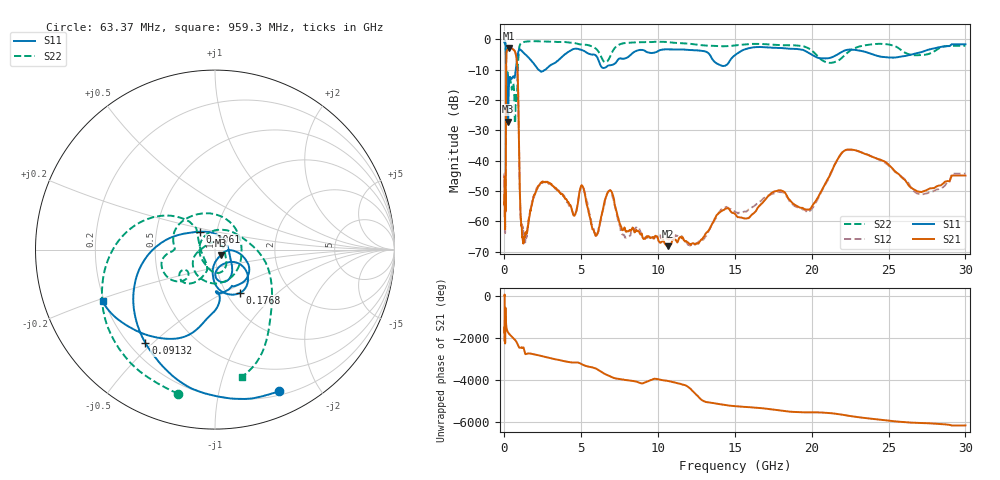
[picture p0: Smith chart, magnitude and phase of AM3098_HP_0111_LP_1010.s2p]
! Date/Time: Thu, Feb 28, 2019 8:39 AM
! Network Analyzer: Agilent Technologies E8364B Rev: A.07.50.67
! Sweep from 0.010 to 30.000 GHz, 1601 Points, Sweep Type: LOG
! Power Supply: 5.022 V, 0.002 A
# Hz S DB R 50
!freq MagS11 AngS11 MagS21 AngS21 MagS12 AngS12 MagS22 AngS22
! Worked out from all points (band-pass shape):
!   1601 points, 10 MHz to 30 GHz, reference 50 ohm
!   highest |S21| = -2.82 dB at 293 MHz (marker M1); lowest = -68.2 dB at 10.65 GHz (marker M2)
!   |S21| within 3 dB of the highest: 121.8 MHz to 773.3 MHz (651.4 MHz wide, 146 % of centre)
!   lowest |S11| = -27.1 dB at 239.9 MHz (marker M3), VSWR 1.09, Z = 53.3 - j3.15 ohm
!   |S11| at or under -10 dB: 102.2 MHz to 730.8 MHz (628.6 MHz wide, 151 % of centre); 2.223 GHz to 2.656 GHz (433.5 MHz wide, 17.8 % of centre)
!   |S22| runs from -27.7 to -0.6 dB; largest |S21 - S12| = 0.01
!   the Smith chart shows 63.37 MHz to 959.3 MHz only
!   S11 on the Smith chart (normalised r, x): 63.37 MHz: 0.24, -1.52; 91.32 MHz: 0.26, -0.47; 106.1 MHz: 0.83, +0.17; 176.8 MHz: 1.15, -0.60; 959.3 MHz: 0.19, -0.21
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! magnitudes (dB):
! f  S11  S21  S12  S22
! 10 MHz  -0.3  -45.2  -44.6  -0.6
! 38.04 MHz  -0.5  -60.3  -59.6  -0.9
! 63.37 MHz  -1.2  -51.4  -51.4  -1.6
! 91.32 MHz  -3.8  -44.4  -42.7  -4.1
! 106.1 MHz  -17.7  -13.5  -13.5  -21.3
! 144.7 MHz  -19.8  -4.0  -4.0  -14.2
! 176.8 MHz  -11.1  -3.5  -3.5  -10.2
! 239.9 MHz  -27.1  -2.9  -2.9  -12.5
! 293 MHz  -14.9  -2.8  -2.8  -12.6
! 550.5 MHz  -12.3  -3.3  -3.2  -14.6
! 825.6 MHz  -6.3  -8.5  -8.5  -17.9
! 959.3 MHz  -3.2  -38.6  -39.0  -2.8
! 1.196 GHz  -4.1  -66.3  -62.1  -0.9
! 2.084 GHz  -9.2  -49.6  -49.1  -0.6
! 5.077 GHz  -3.6  -48.3  -48.3  -1.7
! 5.929 GHz  -5.2  -64.8  -63.4  -2.9
! 6.855 GHz  -8.5  -49.8  -49.8  -5.9
! 7.926 GHz  -6.1  -63.4  -65.4  -1.1
! 10.65 GHz  -3.3  -68.2  -65.7  -0.9
! 19.61 GHz  -3.9  -56.0  -56.5  -2.5
! 22.56 GHz  -3.4  -36.3  -36.4  -3.5
! 30 GHz  -1.6  -44.9  -44.3  -2.1
